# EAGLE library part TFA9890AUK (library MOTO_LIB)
Audio Power amplifier
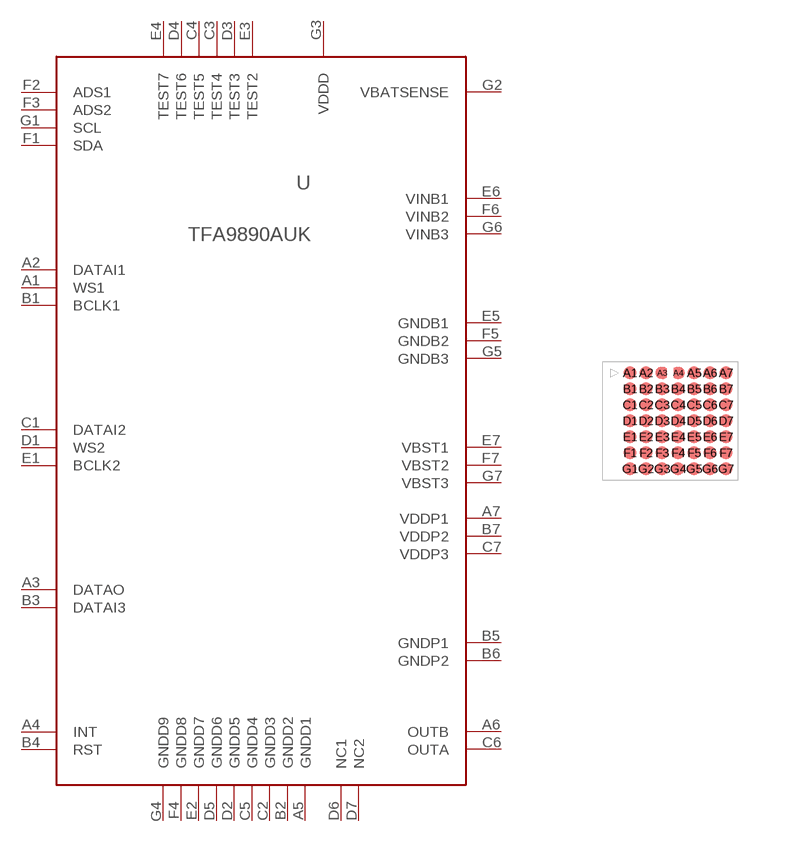
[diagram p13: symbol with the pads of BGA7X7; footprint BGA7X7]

Designator prefix U

## TFA9890AUK (MPN: TFA9890AUK; SUPPLIER: NXP)  [BGA7X7]
A1  WS1
A2  DATAI1
A3  DATAO
A4  INT
A5  GNDD1
A6  OUTB
A7  VDDP1
B1  BCLK1
B2  GNDD2
B3  DATAI3
B4  RST
B5  GNDP1
B6  GNDP2
B7  VDDP2
C1  DATAI2
C2  GNDD3
C3  TEST4
C4  TEST5
C5  GNDD4
C6  OUTA
C7  VDDP3
D1  WS2
D2  GNDD5
D3  TEST3
D4  TEST6
D5  GNDD6
D6  NC1
D7  NC2
E1  BCLK2
E2  GNDD7
E3  TEST2
E4  TEST7
E5  GNDB1
E6  VINB1
E7  VBST1
F1  SDA
F2  ADS1
F3  ADS2
F4  GNDD8
F5  GNDB2
F6  VINB2
F7  VBST2
G1  SCL
G2  VBATSENSE
G3  VDDD
G4  GNDD9
G5  GNDB3
G6  VINB3
G7  VBST3

## Footprint BGA7X7 (pad centres in mm)
smd 0.32 x 0.32: A1 -1,1.2; A2 -0.6,1.2; A5 0.6,1.2; A6 1,1.2; A7 1.4,1.2; B1 -1,0.8; B2 -0.6,0.8; B3 -0.2,0.8; B4 0.2,0.8; B5 0.6,0.8; B6 1,0.8; B7 1.4,0.8; C1 -1,0.4; C2 -0.6,0.4; C3 -0.2,0.4; C4 0.2,0.4; C5 0.6,0.4; C6 1,0.4; C7 1.4,0.4; D1 -1,0; D2 -0.6,0; D3 -0.2,0; D4 0.2,0; D5 0.6,0; D6 1,0; D7 1.4,0; E1 -1,-0.4; E2 -0.6,-0.4; E3 -0.2,-0.4; E4 0.2,-0.4; E5 0.6,-0.4; E6 1,-0.4; E7 1.4,-0.4; F1 -1,-0.8; F2 -0.6,-0.8; F3 -0.2,-0.8; F4 0.2,-0.8; F5 0.6,-0.8; F6 1,-0.8; F7 1.4,-0.8; G1 -1,-1.2; G2 -0.6,-1.2; G3 -0.2,-1.2; G4 0.2,-1.2; G5 0.6,-1.2; G6 1,-1.2; G7 1.4,-1.2
smd 0.22 x 0.22: A3 -0.2,1.2; A4 0.2,1.2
